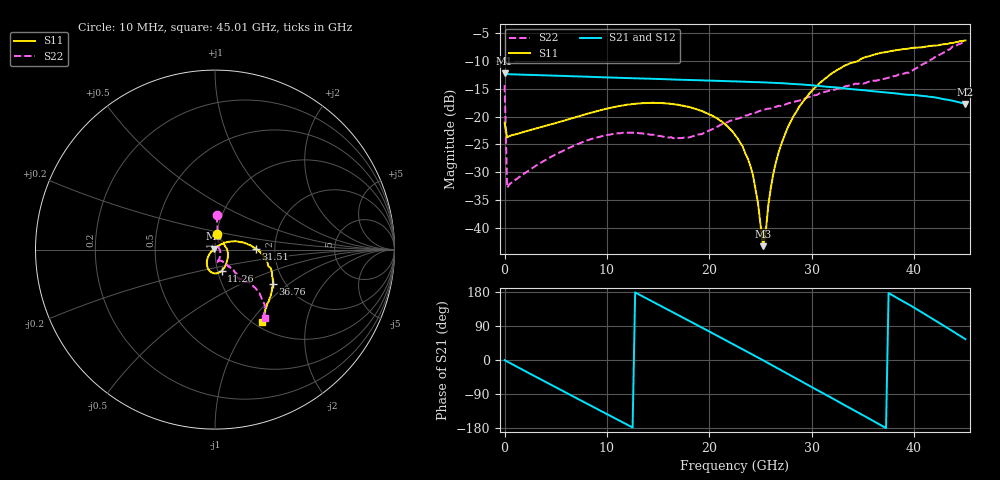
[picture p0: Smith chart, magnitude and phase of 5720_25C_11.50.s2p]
! Device:  ADRF5720
! Description: 0.5dB LSB GaAs MMIC 6-bit Digital Attenuator
! Frequency:  0.000009 -  40 GHz
! Ports:
!	RF1	= Port 1
!	RF2	= Port 2
! Vdd:  3.3 Volt
! Vss:  -3.3 Volt
! Control:  0/3.3 Volt
! State:  11.50 dB attenuation
! Data:  The device was measured using G-S-G Probes on a matrix board.
!  Data was collected using an calibrated 4 port network analyzer.
!  The reference plane for this measurement is at the launchers.
! Note:  Analog Devices supplies this data as a sample of measured data
!  for this product.  Your particular data for this product may vary.
!  Data was taken at 25 degrees C.
!  Analog Devices reserves the right to change this data at anytime.
# GHZ S DB R 45.0
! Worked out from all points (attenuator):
!   181 points, 10 MHz to 45.01 GHz, reference 45 ohm
!   highest |S21| = -12.19 dB at 10 MHz (marker M1); lowest = -17.7 dB at 45.01 GHz (marker M2)
!   lowest |S11| = -43.3 dB at 25.26 GHz (marker M3), VSWR 1.01, Z = 44.5 + j0.407 ohm
!   |S11| at or under -10 dB: start of sweep to 34.54 GHz
!   |S22| runs from -32.8 to -6.5 dB; largest |S21 - S12| = 0.00033
!   S11 on the Smith chart (normalised r, x): 10 MHz: 1.01, +0.18; 11.26 GHz: 1.05, -0.25; 31.51 GHz: 1.59, +0.02; 36.76 GHz: 1.74, -0.77; 45.01 GHz: 1.08, -1.15
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0.01  -21.12 81.8  -12.19 -0.3  -12.19 -0.3  -14.35 87.2
0.26  -23.75 5.9  -12.37 -4.0  -12.38 -4.0  -32.82 19.3
4.26  -21.54 -31.9  -12.61 -61.4  -12.61 -61.4  -27.55 -45.9
7.76  -19.67 -54.1  -12.82 -111.0  -12.82 -111.0  -24.50 -67.3
11.26  -18.10 -72.8  -13.03 -160.5  -13.04 -160.5  -23.02 -80.0
15.26  -17.56 -92.1  -13.26 142.8  -13.26 142.8  -23.53 -83.1
18.01  -18.27 -104.9  -13.43 103.7  -13.43 103.7  -23.78 -69.8
20.26  -19.80 -115.1  -13.55 71.5  -13.55 71.5  -22.30 -58.3
22.76  -23.90 -130.8  -13.69 35.5  -13.70 35.5  -20.40 -53.0
24.26  -30.51 -147.1  -13.79 13.7  -13.80 13.8  -19.44 -52.0
24.76  -35.64 -158.1  -13.81 6.5  -13.82 6.5  -19.11 -51.8
25.26  -43.33 137.9  -13.85 -0.9  -13.85 -0.9  -18.86 -52.0
25.51  -40.82 80.7  -13.87 -4.6  -13.87 -4.5  -18.68 -52.1
26.01  -32.81 52.8  -13.91 -11.9  -13.91 -11.9  -18.54 -51.2
27.01  -25.06 37.4  -14.00 -26.7  -14.00 -26.7  -18.09 -50.1
28.26  -19.83 26.5  -14.14 -45.2  -14.15 -45.2  -17.35 -49.8
30.26  -14.90 10.7  -14.42 -75.1  -14.42 -75.1  -16.19 -48.3
31.51  -12.90 1.4  -14.65 -93.7  -14.65 -93.6  -15.47 -48.6
36.76  -8.54 -30.5  -15.58 -172.2  -15.58 -172.1  -13.32 -49.5
37.76  -8.20 -35.2  -15.76 172.8  -15.76 172.9  -12.97 -47.7
41.76  -7.26 -49.0  -16.48 109.5  -16.48 109.6  -9.67 -44.1
45.01  -6.31 -57.1  -17.73 55.0  -17.74 55.1  -6.48 -53.8
